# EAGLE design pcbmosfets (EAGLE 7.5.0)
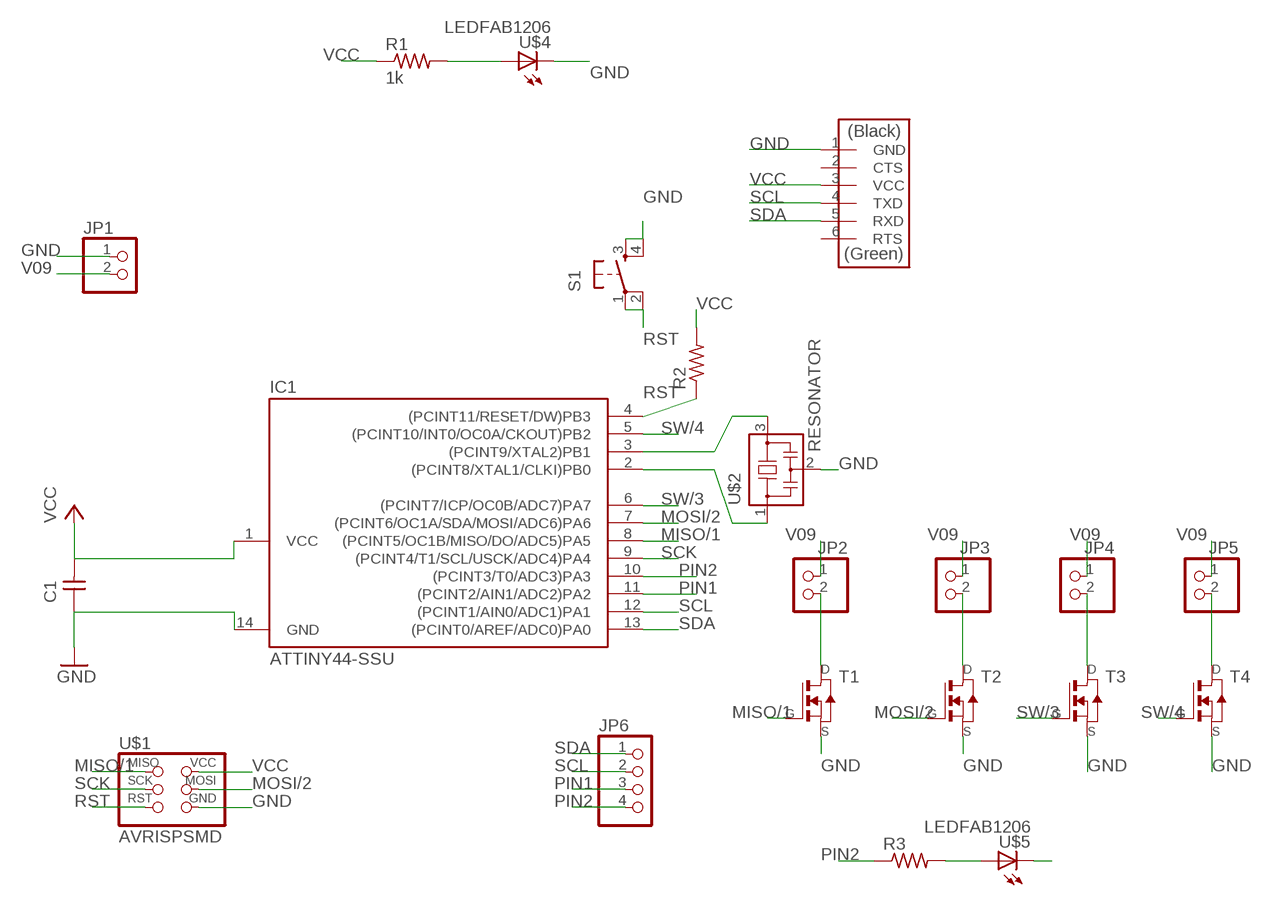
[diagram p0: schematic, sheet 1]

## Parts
C1  CAP-UNPOLARIZEDFAB  [C1206FAB]
IC1  ATTINY44-SSU  [SOIC14]
JP1  PINHD-1X2  [1X02]
JP2  PINHD-1X2  [1X02]
JP3  PINHD-1X2  [1X02]
JP4  PINHD-1X2  [1X02]
JP5  PINHD-1X2  [1X02]
JP6  PINHD-1X4  [1X04]
R1  1k  RES-US1206FAB  [R1206FAB]
R2  RES-US1206FAB  [R1206FAB]
R3  RES-US1206FAB  [R1206FAB]
S1  6MM_SWITCH6MM_SWITCH  [6MM_SWITCH]
T1  NMOSFETSOT23  [SOT-23]
T2  NMOSFETSOT23  [SOT-23]
T3  NMOSFETSOT23  [SOT-23]
T4  NMOSFETSOT23  [SOT-23]
U$1  AVRISPSMD  [2X03SMD]
U$2  RESONATOR  [EFOBM]
U$3  FTDI-SMD-HEADER  [1X06SMD]
U$4  LEDFAB1206  [LED1206FAB]
U$5  LEDFAB1206  [LED1206FAB]

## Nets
GND: C1.1 IC1.14(GND) JP1.1 S1.3(S) S1.4(S1) T1.2(S) T2.2(S) T3.2(S) T4.2(S) U$1.6(GND) U$2.2 U$3.1(GND) U$4.2(C) U$5.2(C)
MISO/1: IC1.8((PCINT5/OC1B/MISO/DO/ADC5)PA5) T1.3(G) U$1.1(MISO)
MOSI/2: IC1.7((PCINT6/OC1A/SDA/MOSI/ADC6)PA6) T2.3(G) U$1.4(MOSI)
N$1: IC1.2((PCINT8/XTAL1/CLKI)PB0) U$2.1
N$2: IC1.3((PCINT9/XTAL2)PB1) U$2.3
N$3: R1.2 U$4.1(A)
N$5: JP2.2 T1.1(D)
N$6: R3.2 U$5.1(A)
N$7: JP5.2 T4.1(D)
N$9: JP3.2 T2.1(D)
N$11: JP4.2 T3.1(D)
PIN1: IC1.11((PCINT2/AIN1/ADC2)PA2) JP6.3
PIN2: IC1.10((PCINT3/T0/ADC3)PA3) JP6.4 R3.1
RST: IC1.4((PCINT11/RESET/DW)PB3) R2.1 S1.1(P) S1.2(P1) U$1.5(RST)
SCK: IC1.9((PCINT4/T1/SCL/USCK/ADC4)PA4) U$1.3(SCK)
SCL: IC1.12((PCINT1/AIN0/ADC1)PA1) JP6.2 U$3.4(TXD)
SDA: IC1.13((PCINT0/AREF/ADC0)PA0) JP6.1 U$3.5(RXD)
SW/3: IC1.6((PCINT7/ICP/OC0B/ADC7)PA7) T3.3(G)
SW/4: IC1.5((PCINT10/INT0/OC0A/CKOUT)PB2) T4.3(G)
V09: JP1.2 JP2.1 JP3.1 JP4.1 JP5.1
VCC: C1.2 IC1.1(VCC) R1.1 R2.2 U$1.2(VCC) U$3.3(VCC)
Unconnected: U$3.2(CTS) U$3.6(RTS)

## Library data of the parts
C1 = fab:CAP-UNPOLARIZED
IC1 = fab:ATTINY44
JP1-JP5 = pinhead:PINHD-1X2: PIN HEADER
JP6 = pinhead:PINHD-1X4: PIN HEADER
R1-R3 = fab:RES-US: Resistor (US Symbol)
S1 = fab:6MM_SWITCH: OMRON SWITCH
T1-T4 = fab:NMOSFET: MOS FET
U$1 = fab:AVRISP
U$2 = fab:RESONATOR
U$3 = fab:FTDI-SMD-HEADER
U$4 U$5 = fab:LED: LED

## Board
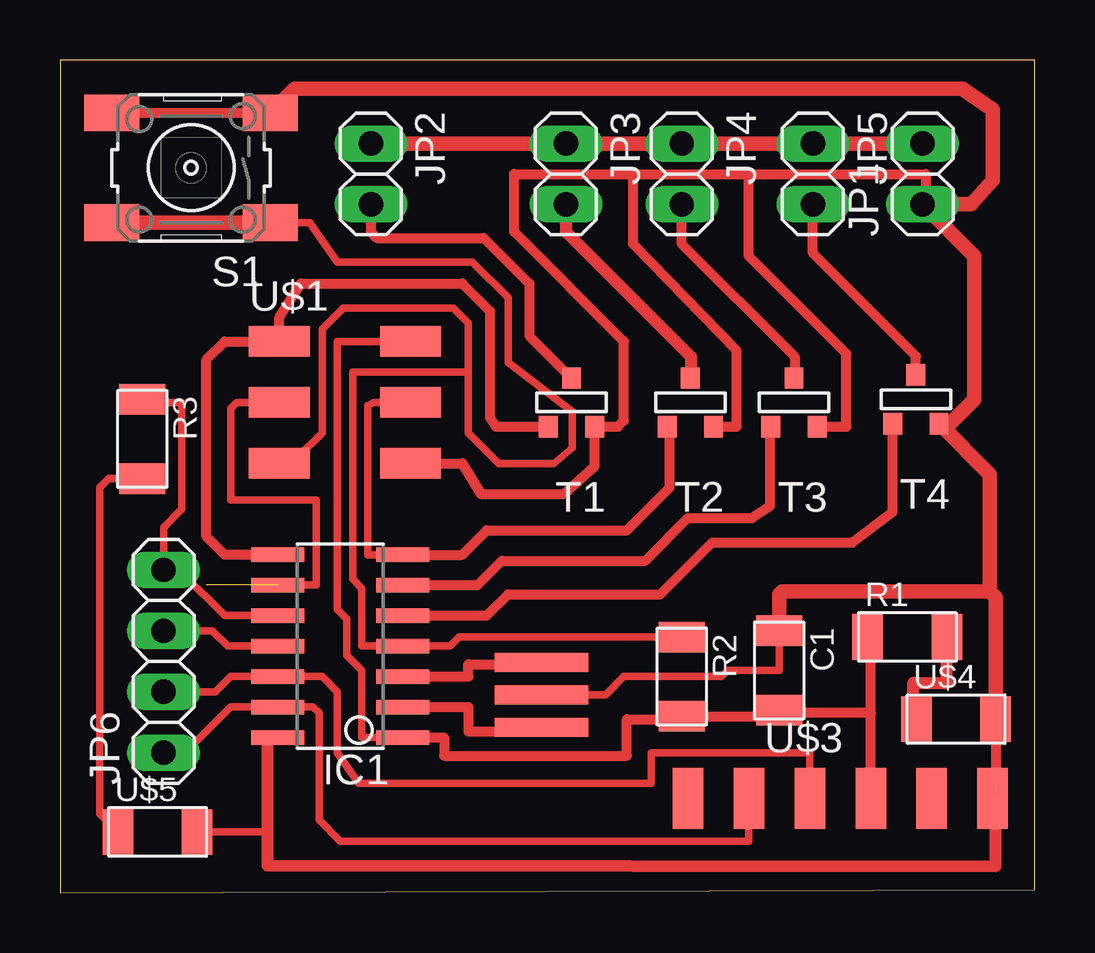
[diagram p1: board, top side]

Size 40.62 x 34.72 mm. Coordinates in mm from the lower left corner, seen from the top.
Outline: 0,0 40.62,0.13 40.62,34.72 0,34.72 0,0
Copper layers (1*16): Top 0.035mm / dielectric 1.5mm / Bottom 0.035mm
Design rules "default *": minimum track width 10mil, minimum drill 24mil, track to track 12mil, track to pad 12mil, pad to pad 12mil, via to via 12mil, smd to smd 12mil, copper to edge 40mil, drill to drill 8mil, minimum pad ring 10mil, minimum via ring 8mil, stop-mask expansion 4mil, vias tented up to drill 0mil, thermal gap 10mil

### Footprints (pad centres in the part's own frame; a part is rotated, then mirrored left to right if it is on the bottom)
C1206FAB = smd 1.27 x 1.905: 1 -1.651,0; 2 1.651,0
SOIC14 = smd 0.61 x 2.21: 1 -3.81,-2.603; 2 -2.54,-2.603; 3 -1.27,-2.603; 4 0,-2.603; 5 1.27,-2.603; 6 2.54,-2.603; 7 3.81,-2.603; 8 3.81,2.603; 9 2.54,2.603; 10 1.27,2.603; 11 0,2.603; 12 -1.27,2.603; 13 -2.54,2.603; 14 -3.81,2.603
1X02 = drill 1.016 long: 1 -1.27,0; 2 1.27,0
1X04 = drill 1.016 long: 1 -3.81,0; 2 -1.27,0; 3 1.27,0; 4 3.81,0
R1206FAB = smd 1.27 x 1.905: 1 -1.651,0; 2 1.651,0
6MM_SWITCH = smd 2.286 x 1.524: 1 -3.302,2.286; 2 3.302,2.286; 3 -3.302,-2.286; 4 3.302,-2.286
SOT-23 = smd 0.787 x 0.889: 1 0.025,-1.016; 2 -0.94,1.016; 3 0.991,1.016
2X03SMD = smd 2.54 x 1.27: 1 -2.54,2.54; 2 2.92,2.54; 3 -2.54,0; 4 2.92,0; 5 -2.54,-2.54; 6 2.92,-2.54
EFOBM = smd 0.8 x 3.9: 1 -1.35,0; 2 0,0; 3 1.35,0
1X06SMD = smd 2.54 x 1.27: 1 0,6.35; 2 0,3.81; 3 0,1.27; 4 0,-1.27; 5 0,-3.81; 6 0,-6.35
LED1206FAB = smd 1.27 x 1.905: 1 -1.651,0; 2 1.651,0

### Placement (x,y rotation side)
C1  29.97,9.27 270 top
IC1  11.68,10.29 90 top
JP1  35.94,29.97 90 top
JP2  12.95,29.97 270 top
JP3  21.08,29.97 270 top
JP4  25.91,29.97 270 top
JP5  31.37,29.97 270 top
JP6  4.32,9.65 90 top
R1  35.31,10.67 0 top
R2  25.91,9.02 270 top
R3  3.43,18.92 270 top
S1  5.46,30.23 180 top
T1  21.34,20.45 180 top
T2  26.29,20.45 180 top
T3  30.61,20.45 180 top
T4  35.69,20.57 180 top
U$1  11.68,20.45 0 top
U$2  20.07,8.25 90 top
U$3  32.51,3.94 270 top
U$4  37.34,7.24 0 top
U$5  4.06,2.54 0 top

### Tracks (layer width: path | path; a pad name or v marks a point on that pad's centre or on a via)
GND  (1 unrouted)
  Top 0.305: U$2.2 22.73,8.25 23.5,9.02 27.56,9.02 27.81,9.27 29.97,9.27 C1.1 | U$5.2 8.51,2.54 8.64,2.41
  Top 0.406: IC1.14 8.64,6.48 | S1.3 S1.4 | U$1.6 16.76,17.91 17.53,16.64 21.01,16.64 22.28,17.78 T1.2 23.24,19.43 23.5,19.68 23.5,22.99 18.92,27.56 18.92,29.97 24,29.97 | 24,29.97 28.7,29.97 | 28.7,29.97 36.07,29.97 36.07,28.83 | T2.2 28.19,19.43 28.19,22.61 23.88,27.05 23.88,29.85 24,29.97 | T3.2 32.77,19.43 32.77,22.48 28.7,26.54 28.7,29.97 | U$4.2 38.99,4.44 | 38.99,3.81 U$3.1
  Top 0.508: 8.64,6.48 8.64,2.41 8.64,1.14 38.99,1.12 38.99,3.81
  Top 0.61: 38.99,4.06 U$3.1 | C1.1 29.97,12.45 30.1,12.57 38.73,12.57 | 38.73,12.57 38.73,17.45 T4.2 37.08,19.56 38.1,20.57 38.1,26.54 JP1.1 | S1.3 9.78,33.53 37.59,33.53 38.86,32.64 38.86,29.72 37.97,28.7 JP1.1 | U$4.2 38.99,12.32 38.73,12.57 | 36.07,28.83 JP1.1
MISO/1
  Top 0.406: IC1.8 6.86,14.1 6.1,14.86 6.1,22.22 6.86,22.99 U$1.1 9.14,24 10.03,25.4 16.76,25.4 17.91,24.26 17.91,19.81 18.16,19.43 T1.3
MOSI/2
  Top 0.305: U$1.4 13.08,20.45 12.83,20.32 12.83,14.1 IC1.7
  Top 0.406: IC1.7 16.76,14.1 17.78,15.11 23.62,15.11 25.4,16.89 25.4,19.2 T2.3
N$1
  Top 0.406: IC1.2 17.02,7.75 17.02,6.73 20.07,6.73 U$2.1
N$2
  Top 0.406: IC1.3 17.02,9.02 17.02,9.53 20.07,9.53 U$2.3
N$3
  Top 0.508: U$4.1 35.56,7.24 35.56,8.76 36.96,8.76 R1.2
N$5
  Top 0.406: JP2.2 12.95,27.56 13.21,27.3 17.65,27.3 19.56,25.4 19.56,23.22 T1.1
N$6
  Top 0.305: R3.2 2.03,17.27 1.65,16.89 1.65,3.3 U$5.1
N$7
  Top 0.406: T4.1 35.66,22.38 31.37,26.67 JP5.2
N$9
  Top 0.508: JP3.2 21.08,27.56 26.29,22.35 26.29,21.49 T2.1
N$11
  Top 0.406: JP4.2 25.91,27.05 30.61,22.35 30.61,21.49 T3.1
PIN1
  Top 0.305: IC1.11 6.98,10.29 6.35,10.92 JP6.3
PIN2
  Top 0.305: IC1.10 6.86,11.56 5.08,13.33 4.45,13.33 JP6.4 4.32,15.24 5.08,16 5.08,20.45 3.56,20.45 R3.1
RST
  Top 0.305: 17.02,21.72 12.19,21.72 12.19,13.08 12.57,12.7 12.57,10.29 IC1.4 16.26,10.29 16.64,10.67 R2.1 | 17.02,21.72 17.02,19.18 18.29,17.91 20.57,17.91 21.34,18.54 21.34,20.07 18.67,22.1 18.67,24.81 17.19,26.29 11.56,26.29 10.41,27.94 S1.1 | U$1.5 9.4,18.16 9.91,18.16 10.92,19.18 10.92,23.5 11.81,24.38 16.38,24.38 17.02,23.75 17.02,21.72
  Top 0.406: 25.91,10.29 R2.1
  Top 0.61: S1.2 S1.1
SCK  (1 unrouted)
  Top 0.305: U$1.3 7.37,20.45 7.11,20.19 7.11,16.38 10.67,16.38 10.67,12.83 IC1.9
SCL
  Top 0.305: U$3.4 31.24,5.84 24.64,5.84 24.64,4.57 12.45,4.57 11.56,5.84 11.56,8.38 10.92,9.02 IC1.12 7.11,9.02 6.48,8.38 JP6.2
SDA
  Top 0.305: U$3.5 28.7,2.16 11.68,2.16 10.8,3.05 10.8,7.49 10.54,7.75 IC1.13 7.11,7.75 5.21,5.84 JP6.1
SW/3
  Top 0.406: IC1.6 17.4,12.83 18.41,13.84 24.38,13.84 26.16,15.62 28.83,15.62 29.59,16.13 29.59,19.15 T3.3
SW/4
  Top 0.406: IC1.5 17.78,11.56 18.67,12.45 25.02,12.45 27.18,14.61 33.02,14.61 34.7,15.87 T4.3
V09
  Top 0.61: JP1.2 JP5.1 JP4.1 JP3.1 JP2.1
VCC
  Top 0.305: U$1.2 11.56,22.99 11.56,11.81 11.94,11.43 11.94,9.91 12.57,9.27 12.57,6.48 IC1.1
  Top 0.406: IC1.1 16,6.48 16,5.71 23.62,5.71 23.62,7.24 25.91,7.24 R2.2 29.97,7.37 C1.2 29.97,7.49 33.78,7.49 | U$3.3 33.78,7.49 | 33.78,7.49 33.78,10.54 R1.1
